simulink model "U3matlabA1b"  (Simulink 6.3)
settings: Solver=ode45  StartTime=0.0  StopTime=10.0  RelTol=1e-3
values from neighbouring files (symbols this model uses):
  A = [-1 3 2; -5 -2 1;-2 3 -1]    [U3muloe.m]
  b = [-1; 3; 1]    [U3muloe.m]
  c = [1 .5 3]    [U3muloe.m]
  d = .1    (= 0.1)    [U3muloe.m]

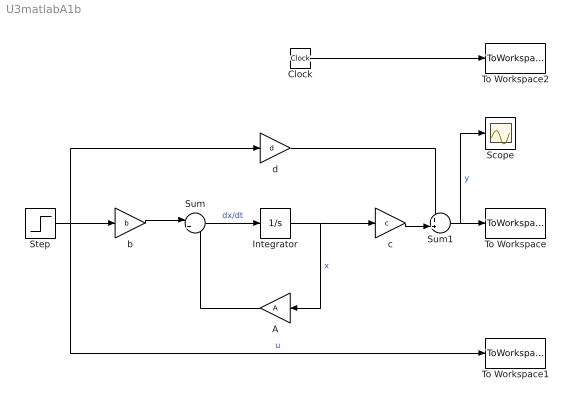
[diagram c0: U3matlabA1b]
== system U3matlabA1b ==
  A : Gain  Orientation=left  Gain=A  Multiplication=Matrix(K*u)
  Clock : Clock
  Integrator : Integrator
  Scope : Scope
  Step : Step  SampleTime=0
  Sum : Sum  Inputs=|++
  Sum1 : Sum  Inputs=++|
  To Workspace : ToWorkspace  VariableName=y  SampleTime=-1  SaveFormat=Array
  To Workspace1 : ToWorkspace  VariableName=u  SampleTime=-1  SaveFormat=Array
  To Workspace2 : ToWorkspace  VariableName=t  SampleTime=-1  SaveFormat=Array
  b : Gain  Gain=b  Multiplication=Matrix(K*u)
  c : Gain  Gain=c  Multiplication=Matrix(K*u)
  d : Gain  Gain=d  Multiplication=Matrix(K*u)
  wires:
  Step/1 -> b/1, To Workspace1/1, d/1  "u"
  b/1 -> Sum/1
  Sum/1 -> Integrator/1  "dx/dt"
  Integrator/1 -> c/1, A/1  "x"
  A/1 -> Sum/2
  Clock/1 -> To Workspace2/1
  Sum1/1 -> To Workspace/1, Scope/1  "y"
  c/1 -> Sum1/2
  d/1 -> Sum1/1
